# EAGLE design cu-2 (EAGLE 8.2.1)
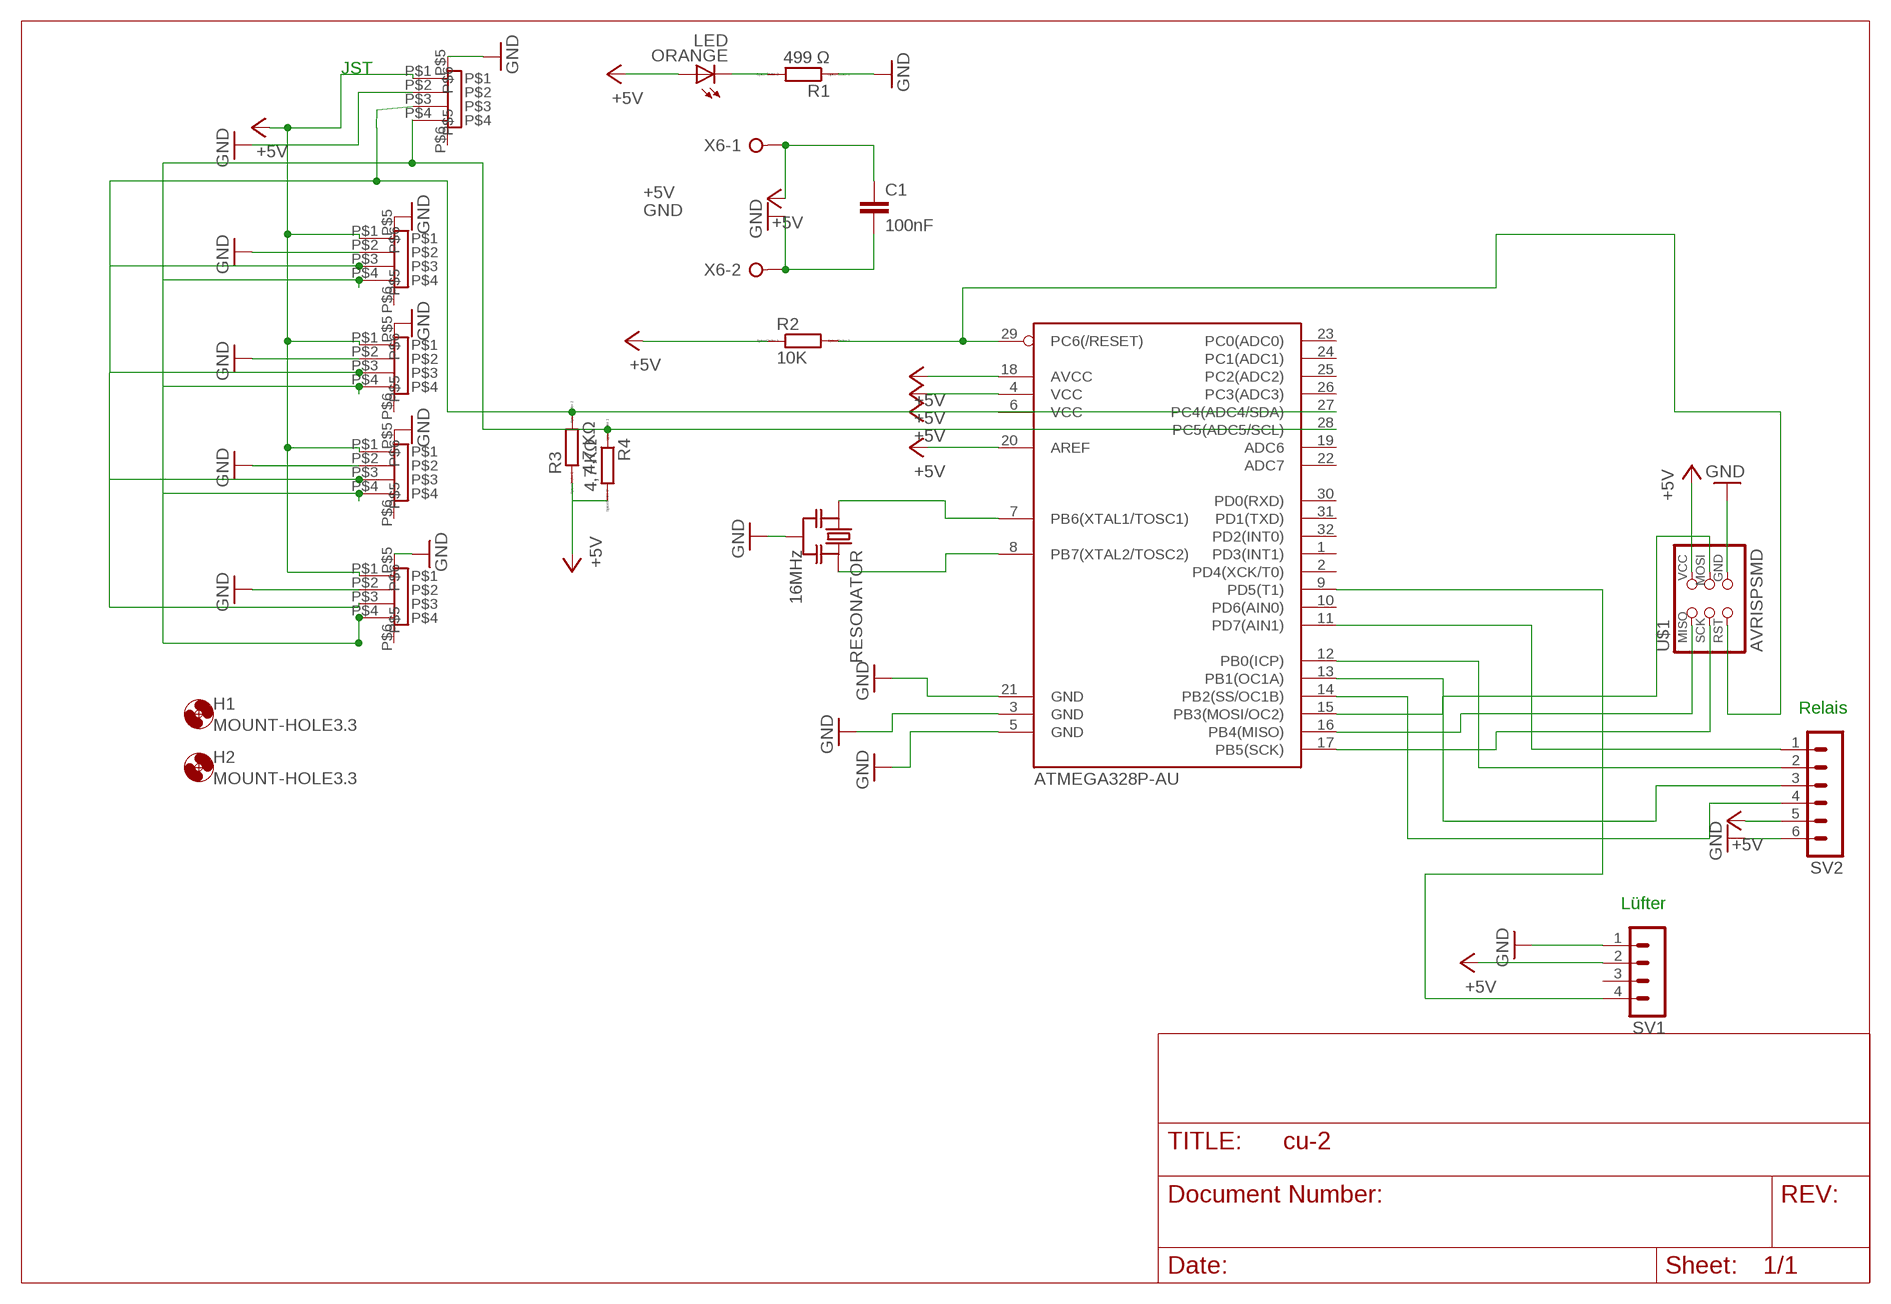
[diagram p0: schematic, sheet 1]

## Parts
ATMEGA328P-AU  ATMEGA88-THIN  [TQFP32-08THIN]
C1  100nF  C-EUC1206  [C1206]
H1  MOUNT-HOLE3.3  [3,3]
H2  MOUNT-HOLE3.3  [3,3]
ORANGE  LED  [LED1206]
R1  499 Ω  RR1206  [R1206]
R2  10K  RR1206  [R1206]
R3  4,7 KΩ  RR1206  [R1206]
R4  4,7 KΩ  RR1206  [R1206]
RESONATOR  16MHz  RESONATOR-MURATACSTCR_G  [RESONATOR_MURATA3]
SV1  MA04-1  [MA04-1]
SV2  MA06-1  [MA06-1]
U$1  AVRISPSMD  [2X03SMD]
U$2  PHP4_SM4  [PH4P_SM4]
U$3  PHP4_SM4  [PH4P_SM4]
U$4  PHP4_SM4  [PH4P_SM4]
U$5  PHP4_SM4  [PH4P_SM4]
U$6  PHP4_SM4  [PH4P_SM4]
X6  W237-02P  [W237-132]

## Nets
+5V: ATMEGA328P-AU.4(VCC) ATMEGA328P-AU.6(VCC) ATMEGA328P-AU.18(AVCC) ATMEGA328P-AU.20(AREF) C1.1 ORANGE.1(A) R2.1 R3.1 R4.2 SV1.2 SV2.5 U$1.2(VCC) U$2.P$1 U$3.P$1 U$4.P$1 U$5.P$1 U$6.P$1 X6.1
GND: ATMEGA328P-AU.3(GND) ATMEGA328P-AU.5(GND) ATMEGA328P-AU.21(GND) C1.2 R1.1 RESONATOR.2 SV1.1 SV2.6 U$1.6(GND) U$2.P$2 U$2.P$5 U$3.P$2 U$3.P$5 U$4.P$2 U$4.P$5 U$5.P$2 U$5.P$5 U$6.P$2 U$6.P$5 X6.2
N$1: ATMEGA328P-AU.11(PD7(AIN1)) SV2.1
N$2: ATMEGA328P-AU.12(PB0(ICP)) SV2.2
N$3: ATMEGA328P-AU.13(PB1(OC1A)) SV2.3
N$4: ATMEGA328P-AU.14(PB2(SS/OC1B)) SV2.4
N$6: ATMEGA328P-AU.15(PB3(MOSI/OC2)) U$1.4(MOSI)
N$13: ATMEGA328P-AU.9(PD5(T1)) SV1.4
N$19: ATMEGA328P-AU.17(PB5(SCK)) U$1.3(SCK)
N$20: ATMEGA328P-AU.16(PB4(MISO)) U$1.1(MISO)
N$24: ORANGE.2(C) R1.2
N$27: ATMEGA328P-AU.7(PB6(XTAL1/TOSC1)) RESONATOR.1
N$28: ATMEGA328P-AU.8(PB7(XTAL2/TOSC2)) RESONATOR.3
N$29: ATMEGA328P-AU.29(PC6(/RESET)) R2.2 U$1.5(RST)
SCL: ATMEGA328P-AU.28(PC5(ADC5/SCL)) R4.1 U$2.P$4 U$3.P$4 U$4.P$4 U$5.P$4 U$6.P$4
SDA: ATMEGA328P-AU.27(PC4(ADC4/SDA)) R3.2 U$2.P$3 U$3.P$3 U$4.P$3 U$5.P$3 U$6.P$3
Unconnected: ATMEGA328P-AU.1(PD3(INT1)) ATMEGA328P-AU.2(PD4(XCK/T0)) ATMEGA328P-AU.10(PD6(AIN0)) ATMEGA328P-AU.19(ADC6) ATMEGA328P-AU.22(ADC7) ATMEGA328P-AU.23(PC0(ADC0)) ATMEGA328P-AU.24(PC1(ADC1)) ATMEGA328P-AU.25(PC2(ADC2)) ATMEGA328P-AU.26(PC3(ADC3)) ATMEGA328P-AU.30(PD0(RXD)) ATMEGA328P-AU.31(PD1(TXD)) ATMEGA328P-AU.32(PD2(INT0)) SV1.3 U$2.P$6 U$3.P$6 U$4.P$6 U$5.P$6 U$6.P$6

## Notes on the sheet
- JST
- Relais
- Lüfter

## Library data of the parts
ATMEGA328P-AU = fab:ATMEGA88-THIN
C1 = rcl:C-EU: CAPACITOR, European symbol
H1 H2 = holes:MOUNT-HOLE: MOUNTING HOLE with drill center marker
ORANGE = fab:LED: LED
R1-R4 = eagle-ltspice:R: RESISTOR, European symbol; SPICEMODEL: NONE; SPICEPREFIX: R
RESONATOR = m-pad-2.1:RESONATOR-MURATA: Murata ceramic Resonator "ceralock" CSTCE series with built in load capacitance +- 0.5% tolerance 12.51MHz to 19.99MHz 16MHz murata part#: CSTCE16M0V53-R0 16MHz digikey part#: 490-1198-1-ND $1.33 each
SV1 = con-lstb:MA04-1: PIN HEADER; OC_FARNELL: unknown; OC_NEWARK: unknown
SV2 = con-lstb:MA06-1: PIN HEADER; OC_FARNELL: unknown; OC_NEWARK: unknown
U$1 = fab:AVRISP
U$2-U$6 = jst_ph_topo:PHP4_SM4
X6 = con-wago-508:W237-02P: WAGO SREW CLAMP; OC_FARNELL: unknown; OC_NEWARK: unknown

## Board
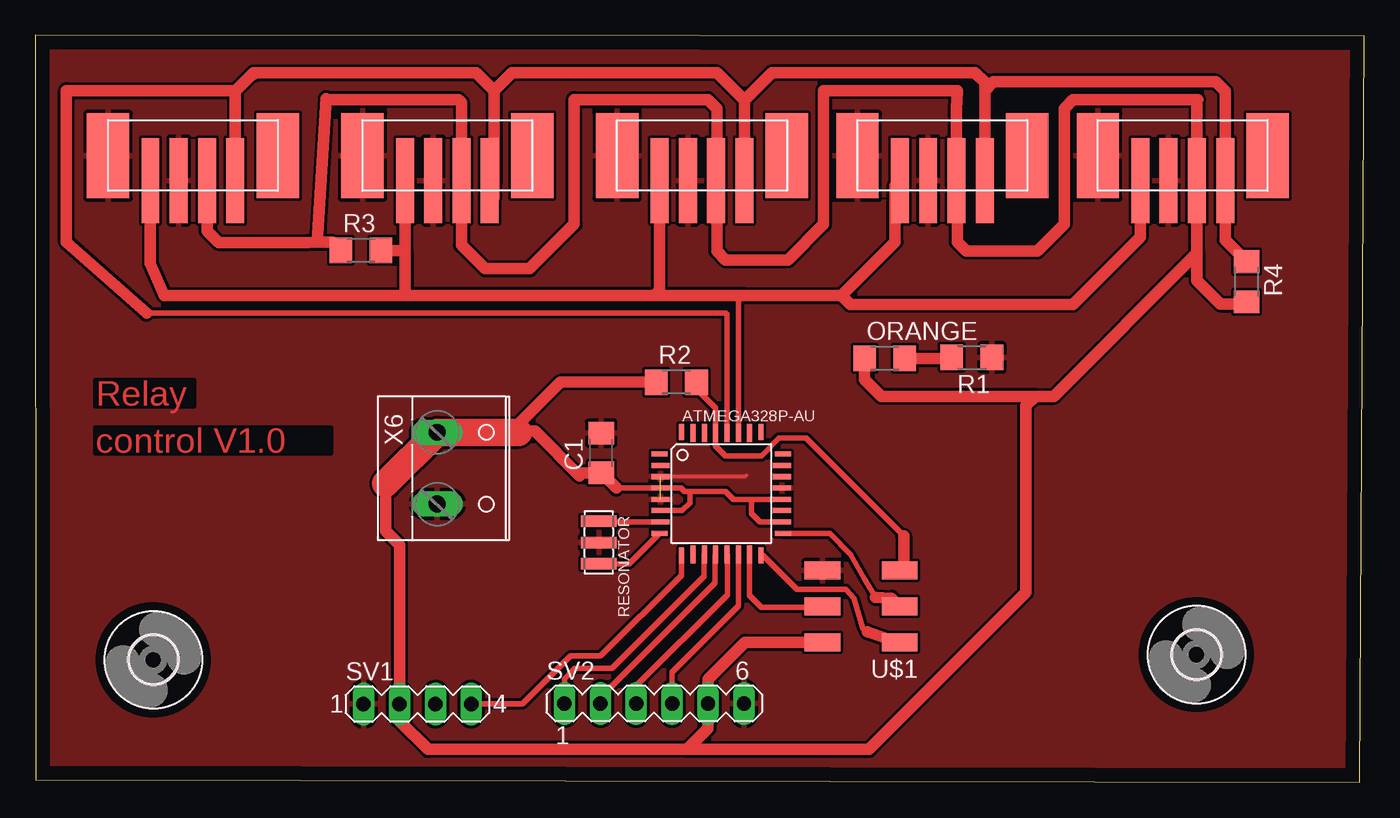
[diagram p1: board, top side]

Size 93.97 x 52.85 mm. Coordinates in mm from the lower left corner, seen from the top.
Outline: 0.03,0.19 93.66,0 93.97,52.77 0,52.85 0.03,0.19
Copper layers (1*16): Top 0.035mm / dielectric 1.5mm / Bottom 0.035mm
Design rules "default": minimum track width 10mil, minimum drill 24mil, track to track 8mil, track to pad 8mil, pad to pad 8mil, via to via 8mil, smd to smd 8mil, copper to edge 40mil, drill to drill 8mil, minimum pad ring 10mil, minimum via ring 8mil, stop-mask expansion 4mil, vias tented up to drill 0mil, thermal gap 10mil

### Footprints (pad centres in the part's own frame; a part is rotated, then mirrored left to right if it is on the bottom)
TQFP32-08THIN = smd 1.118 x 0.356: 1 -4.369,2.8; 8 -4.369,-2.8; 17 4.369,-2.8; 24 4.369,2.8 | smd 1.27 x 0.356: 2 -4.293,2; 3 -4.293,1.2; 4 -4.293,0.4; 5 -4.293,-0.4; 6 -4.293,-1.2; 7 -4.293,-2; 18 4.293,-2; 19 4.293,-1.2; 20 4.293,-0.4; 21 4.293,0.4; 22 4.293,1.2; 23 4.293,2 | smd 0.356 x 1.118: 9 -2.8,-4.369; 16 2.8,-4.369; 25 2.8,4.369; 32 -2.8,4.369 | smd 0.356 x 1.27: 10 -2,-4.293; 14 1.2,-4.293; 15 2,-4.293; 26 2,4.293; 27 1.2,4.293; 31 -2,4.293 | smd 0.35 x 1.27: 11 -1.2,-4.293; 12 -0.4,-4.293; 13 0.4,-4.293; 28 0.4,4.293; 29 -0.4,4.293; 30 -1.2,4.293
C1206 = smd 1.6 x 1.8: 1 -1.4,0; 2 1.4,0
3,3 = hole 3.3: 0,0
LED1206 = smd 1.6 x 1.803: 1 -1.422,0; 2 1.422,0
R1206 = smd 1.6 x 1.803: 1 -1.422,0; 2 1.422,0
RESONATOR_MURATA3 = smd 0.8 x 2.5: 1 -1.5,0; 2 0,0; 3 1.5,0
MA04-1 = drill 1.016 long: 1 -3.81,0; 2 -1.27,0; 3 1.27,0; 4 3.81,0
MA06-1 = drill 1.016 long: 1 -6.35,0; 2 -3.81,0; 3 -1.27,0; 4 1.27,0; 5 3.81,0; 6 6.35,0
2X03SMD = smd 2.54 x 1.27: 1 -2.54,2.54; 2 2.92,2.54; 3 -2.54,0; 4 2.92,0; 5 -2.54,-2.54; 6 2.92,-2.54
PH4P_SM4 = smd 6 x 1.27: P$1 2,2; P$2 2,4; P$3 2,6; P$4 2,0 | smd 6 x 3: P$5 3.75,9; P$6 3.75,-3
W237-132 = drill 1.194 long: 1 -2.54,-0.635; 2 2.54,-0.635

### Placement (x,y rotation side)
ATMEGA328P-AU  48.51,20.43 0 top
C1  40.01,23.31 90 top
H1  82.12,9.04 0 top
H2  8.35,8.68 0 top
ORANGE  60.06,30 0 top
R1  66.22,30.06 180 top
R2  45.33,28.32 0 top
R3  23.02,37.62 0 top
R4  85.66,35.42 270 top
RESONATOR  39.85,16.97 270 top
SV1  27.02,5.54 0 top
SV2  43.76,5.59 0 top
U$1  58.59,12.45 180 top
U$2  84.14,40.58 90 top
U$3  50.14,40.58 90 top
U$4  67.14,40.58 90 top
U$5  14.14,40.58 90 top
U$6  32.14,40.58 90 top
X6  29.05,22.23 270 top

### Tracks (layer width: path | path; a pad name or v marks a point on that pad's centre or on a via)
+5V
  Top 0.406: 50.62,20.03 ATMEGA328P-AU.20 | 50.62,20.03 49.38,20.03 48.82,20.59 46.2,20.59 | 46.2,20.59 45.89,20.59 45.66,20.82 ATMEGA328P-AU.4 41.09,20.83 | ATMEGA328P-AU.18 51.25,18.43 50.64,19.04 50.64,20.01 50.62,20.03 | ATMEGA328P-AU.6 45.74,19.23 46.29,19.78 46.29,20.49 46.2,20.59 | 38.49,21.69 38.7,21.9 | C1.1 | U$1.2 | 34.25,24.85 33.68,24.85 | SV1.2
  Top 0.813: 19.94,38.21 19.3,38.2 12.95,38.2 12.14,39.01 U$5.P$1 12.28,42.72 | 19.94,38.21 20.57,48.37 20.63,48.31 29.92,48.31 30.14,48.09 U$6.P$1 30.14,38.01 31.81,36.34 34.96,36.34 38.11,39.49 38.11,48.31 47.56,48.31 48.19,47.68 48.19,42.63 U$3.P$1 48.19,42.53 48.19,37.6 48.82,36.97 53.23,36.97 55.75,39.49 55.75,48.94 65.2,48.94 65.14,47.62 U$4.P$1 65.2,42.52 65.2,38.23 65.83,37.6 70.87,37.6 72.76,39.49 72.76,47.68 73.39,48.31 82.21,48.31 82.14,48.24 U$2.P$1 82.14,37.43 | 19.94,38.21 21.02,38.21 R3.1 | C1.1 41.09,20.83 | SV1.2 25.75,8.95 25.75,16.8 24.78,17.77 24.78,21.13 | 38.7,21.9 C1.1 | U$1.2 50.2,9.91 47.57,7.29 SV2.5 47.57,3.81 46.09,2.33 | 38.49,21.69 35.33,24.85 34.25,24.85 34.18,24.77 | R2.1 37.15,28.32 33.68,24.85 | 46.09,2.33 27.77,2.33 25.74,4.36 SV1.2 | 82.14,37.43 82.14,35.49 83.79,33.84 85.51,33.84 R4.2 | ORANGE.1 58.64,28.49 59.82,27.31 70.71,27.31 | 70.71,27.31 72.02,27.31 82.14,37.43 | 46.09,2.33 58.95,2.33 70.05,13.43 70.05,26.66 70.71,27.31
  Top 1.93: 24.78,21.13 X6.1 34.18,24.77
GND  (1 unrouted)
  Top 0.254: ATMEGA328P-AU.3 50.2,21.63 50.28,21.71
  pour Top: 96.99,55.04 -3.08,55.18 -2.75,-4 96.71,-4.33
N$1
  Top 0.406: SV2.1 37.41,7.32 38.15,8.05 40.77,8.05 47.29,14.58 47.29,16.11 ATMEGA328P-AU.11
N$2
  Top 0.406: SV2.2 39.95,6.01 48.05,14.11 48.05,16.07 ATMEGA328P-AU.12
N$3
  Top 0.406: SV2.3 42.49,6.82 48.94,13.27 48.94,16.1 ATMEGA328P-AU.13
N$4
  Top 0.406: SV2.4 45.03,7.79 49.73,12.48 49.73,16.12 ATMEGA328P-AU.14
N$6
  Top 0.406: ATMEGA328P-AU.15 50.51,13.23 51.34,12.4 55.61,12.4 U$1.4
N$13
  Top 0.406: SV1.4 34.46,5.54 37.86,8.94 39.98,8.94 45.69,14.65 45.69,16.04 ATMEGA328P-AU.9
N$19
  Top 0.406: ATMEGA328P-AU.17 56.19,17.63 57.66,16.11 58.64,14.41 59.06,13.69 59.42,13.09
  Top 0.813: 59.42,13.09 60.55,13.03 U$1.3
N$20
  Top 0.406: ATMEGA328P-AU.16 51.46,16.06 53.86,13.66 57.32,13.66 57.89,13.01 58.53,10.87 58.84,10.66 | 61.09,9.88 U$1.1
  Top 0.813: 58.84,10.66 61.09,9.88
N$24
  Top 0.406: 64.74,30 R1.2
  Top 0.813: ORANGE.2 64.74,30
N$27
  Top 0.406: ATMEGA328P-AU.7 39.89,18.43 RESONATOR.1
N$28
  Top 0.406: RESONATOR.3 41.98,15.47 ATMEGA328P-AU.8
N$29
  Top 0.406: 61.42,17.44 54.49,24.37 52.6,24.37 51.34,23.11 48.82,23.11 48.11,23.82 ATMEGA328P-AU.29 48.1,26.48 46.75,27.83 R2.2 | 61.42,15.28 U$1.5
  Top 0.813: 61.42,17.44 61.42,15.28
SCL
  Top 0.406: ATMEGA328P-AU.28 48.91,33.1 48.82,33.19 7.87,33.19
  Top 0.813: 14.14,48.91 U$5.P$4 | 15.11,49.88 14.14,48.91 | 15.11,49.88 15.43,50.2 31.18,50.2 32.44,48.94 | 32.44,48.94 32.44,42.28 | 32.44,41.38 32.44,42.28 | 32.44,42.28 U$6.P$4 | 50.14,48.25 U$3.P$4 | 50.14,48.25 48.19,50.2 33.7,50.2 32.44,48.94 | 67.14,48.94 U$4.P$4 | 67.14,48.94 67.14,49.52 66.46,50.2 52.09,50.2 50.14,48.25 | 67.14,48.94 67.77,49.57 83.47,49.57 84.14,48.9 U$2.P$4 84.14,38.37 R4.1 | 15.52,50.13 15.11,49.88 | 7.87,33.19 2.2,38.23 2.2,48.94 14.11,48.94 14.14,48.91
SDA
  Top 0.406: ATMEGA328P-AU.27 49.71,34.08 50.08,34.45
  Top 0.813: U$5.P$3 8.14,36.7 9.13,34.45 26.14,34.45 | 26.14,37.6 26.14,34.45 | 26.14,37.6 U$6.P$3 | 43.78,34.45 50.08,34.45 57.01,34.45 | 43.78,34.45 26.14,34.45 | 57.01,34.45 60.79,38.23 60.79,42.23 U$4.P$3 | U$2.P$3 78.14,38.57 73.39,33.82 57.64,33.82 57.01,34.45 | 43.78,34.45 44.14,34.81 U$3.P$3 | R3.2 26.11,37.62 26.14,37.6

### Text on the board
Top: Relay | control V1.0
